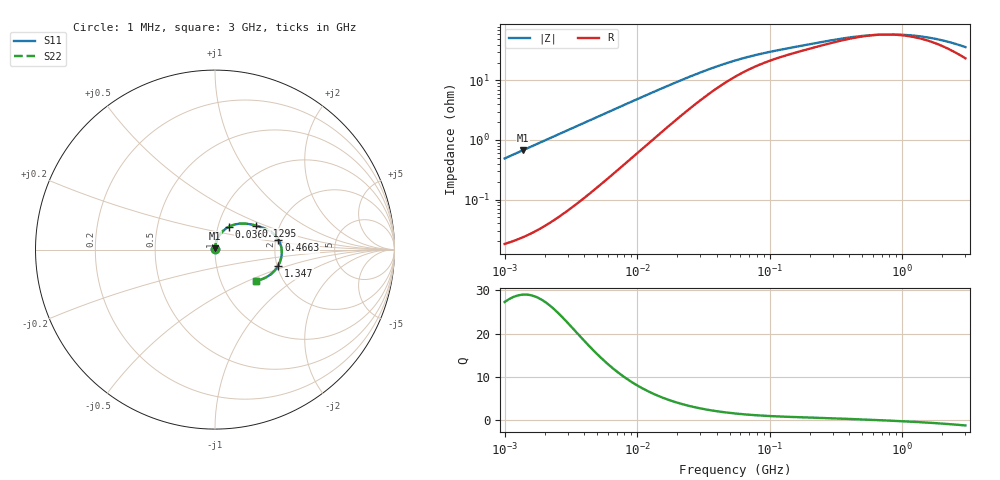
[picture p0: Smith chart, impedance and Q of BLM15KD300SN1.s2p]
! BLM15KD300SN1
# Hz S RI R 50
!Freq.(Hz) S11(Real) S11(Imag) S21(Real) S21(Imag) S12(Real) S12(Imag) S22(Real) S22(Imag)
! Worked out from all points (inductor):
!   401 points, 1 MHz to 3 GHz, reference 50 ohm
!   read as one part in series: L = 77.8 nH near 1.041 MHz
!   highest Q = 28.9 at 1.377 MHz (marker M1), where L = 77.8 nH
!   self-resonance near 720.3 MHz
!   S11 on the Smith chart (normalised r, x): 1 MHz: 1.00, +0.01; 36.7 MHz: 1.13, +0.29; 129.5 MHz: 1.52, +0.44; 466.3 MHz: 2.07, +0.26; 1.347 GHz: 2.03, -0.42; 3 GHz: 1.47, -0.55
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1000000  0.000203 0.00489  0.9998 -0.00489  0.9998 -0.00489  0.000203 0.00489
1040844  0.00021 0.00509  0.9998 -0.00509  0.9998 -0.00509  0.00021 0.00509
1377479  0.000278 0.00673  0.9997 -0.00673  0.9997 -0.00673  0.000278 0.00673
3823119  0.00133 0.0186  0.9987 -0.0186  0.9987 -0.0186  0.00133 0.0186
7858845  0.00517 0.0377  0.9948 -0.0377  0.9948 -0.0377  0.00517 0.0377
1.461624e7  0.0169 0.0671  0.9831 -0.0671  0.9831 -0.0671  0.0169 0.0671
2.41077e7  0.0411 0.1001  0.9589 -0.1001  0.9589 -0.1001  0.0411 0.1001
3.670325e7  0.0785 0.1276  0.9215 -0.1276  0.9215 -0.1276  0.0785 0.1276
5.477226e7  0.1269 0.1432  0.8731 -0.1432  0.8731 -0.1432  0.1269 0.1432
8.011685e7  0.1751 0.1441  0.8249 -0.1441  0.8249 -0.1441  0.1751 0.1441
1.295243e8  0.2291 0.1335  0.7709 -0.1335  0.7709 -0.1335  0.2291 0.1335
2.094008e8  0.2789 0.117  0.7211 -0.117  0.7211 -0.117  0.2789 0.117
3.124888e8  0.3199 0.0933  0.6801 -0.0933  0.6801 -0.0933  0.3199 0.0933
4.66327e8  0.3535 0.0551  0.6465 -0.0551  0.6465 -0.0551  0.3535 0.0551
6.171487e8  0.3677 0.0208  0.6323 -0.0208  0.6323 -0.0208  0.3677 0.0208
8.005644e8  0.3721 -0.0147  0.6279 0.0147  0.6279 0.0147  0.3721 -0.0147
1.038491e9  0.3671 -0.0523  0.6329 0.0523  0.6329 0.0523  0.3671 -0.0523
1.347129e9  0.3515 -0.0902  0.6485 0.0902  0.6485 0.0902  0.3515 -0.0902
1.645649e9  0.3314 -0.1181  0.6686 0.1181  0.6686 0.1181  0.3314 -0.1181
2.050964e9  0.3007 -0.1449  0.6993 0.1449  0.6993 0.1449  0.3007 -0.1449
2.505452e9  0.2656 -0.1633  0.7344 0.1633  0.7344 0.1633  0.2656 -0.1633
3e9  0.2297 -0.1727  0.7703 0.1727  0.7703 0.1727  0.2297 -0.1727
